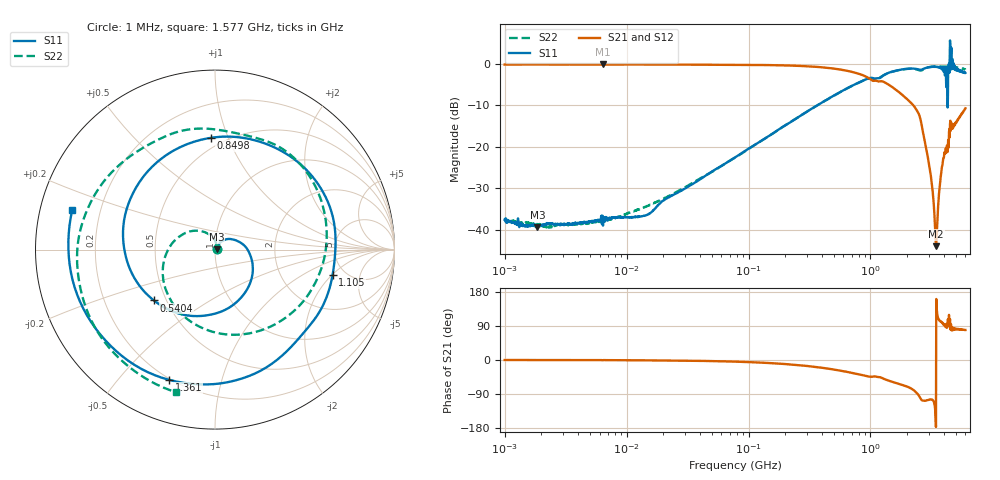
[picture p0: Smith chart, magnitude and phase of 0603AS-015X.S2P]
!s-Parameter Generated by FASTRON Sdn. Bhd.
!FASTRON P/N : 0603AS-015X
!Keysight Technologies: E5071C_MY46733604_B.14.02
!Date: Tue Oct 10 11:21:01 2023
!Version  :Rev01  Tue Oct 10 11:21:01 2023
!Data & Calibration Information:
!Freq  S11:SOLT2(ON)  S21:SOLT2(ON)  S12:SOLT2(ON)  S22:SOLT2(ON)
!PortZ  Port1:50+j0  Port2:50+j0
!When reading reference impedance value at option line is always used.
! Remarks : This data is being provided solely for informational purposes.
# Hz S dB R 50
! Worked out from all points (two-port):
!   1601 points, 1 MHz to 6 GHz, reference 50 ohm
!   highest |S21| = -0.07 dB at 6.378 MHz (marker M1); lowest = -44.0 dB at 3.442 GHz (marker M2)
!   |S21| within 3 dB of the highest: start of sweep to 926.1 MHz
!   lowest |S11| = -39.5 dB at 1.855 MHz (marker M3), VSWR 1.02, Z = 51.1 + j0.174 ohm
!   |S11| at or under -10 dB: start of sweep to 364.6 MHz; 4.290716 GHz to 4.297053 GHz (6.337 MHz wide, 0.148 % of centre)
!   |S22| runs from -39.5 to -0.5 dB; largest |S21 - S12| = 0.005
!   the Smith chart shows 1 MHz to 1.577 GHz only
!   S11 on the Smith chart (normalised r, x): 1 MHz: 1.03, +0.00; 540.4 MHz: 0.43, -0.30; 849.8 MHz: 0.43, +0.87; 1.105 GHz: 3.95, -2.05; 1.361 GHz: 0.19, -0.69; 1.577 GHz: 0.10, +0.14
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1000000  -37.65 7.5  -0.11 -0.0  -0.11 0.0  -37.86 8.2
1855321  -39.48 9.3  -0.11 -0.1  -0.11 -0.1  -38.80 7.3
4277066  -38.35 19.1  -0.11 -0.3  -0.11 -0.3  -38.55 25.3
6378092  -36.69 22.6  -0.07 -0.4  -0.09 -0.4  -37.61 28.8
1.823719e7  -34.04 48.3  -0.11 -1.1  -0.12 -1.0  -33.08 61.0
7.757876e7  -22.56 45.8  -0.16 -4.3  -0.16 -4.3  -22.60 102.9
3.307917e8  -10.76 -53.8  -0.59 -17.2  -0.60 -17.1  -10.77 -168.3
5.404339e8  -7.07 -140.2  -1.23 -26.9  -1.23 -26.9  -7.08 -99.3
8.498359e8  -4.11 92.2  -2.60 -39.6  -2.61 -39.6  -4.13 3.1
1.105144e9  -3.48 -12.3  -4.01 -43.7  -4.02 -43.7  -3.50 89.2
1.36083e9  -2.28 -109.5  -4.71 -52.9  -4.71 -52.7  -2.30 -179.5
1.414819e9  -2.08 -131.0  -5.01 -54.7  -5.01 -54.6  -2.12 -161.0
1.576786e9  -1.67 164.4  -5.95 -59.7  -5.97 -59.6  -1.69 -105.1
1.992454e9  -1.12 1.0  -8.45 -70.2  -8.45 -70.1  -1.16 40.1
2.45304e9  -1.25 -177.2  -11.69 -90.6  -11.70 -90.5  -1.40 -155.9
2.965799e9  -0.81 -10.2  -22.86 -105.7  -22.84 -105.7  -0.78 33.8
3.442219e9  -0.70 166.9  -44.03 -176.8  -44.07 -176.8  -0.54 -155.0
3.847204e9  -1.05 13.2  -24.92 98.7  -24.92 98.6  -0.64 -7.6
4.333184e9  -1.66 -171.3  -18.37 97.4  -18.37 97.1  -0.63 170.5
4.824846e9  -0.15 4.4  -15.08 80.1  -15.09 80.2  -0.69 -9.6
5.608282e9  -1.91 76.3  -11.92 80.3  -11.93 80.4  -1.07 -81.7
6e9  -2.13 -66.5  -10.70 79.1  -10.70 79.2  -1.35 62.5
